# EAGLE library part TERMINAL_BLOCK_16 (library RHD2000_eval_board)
16-point terminal block
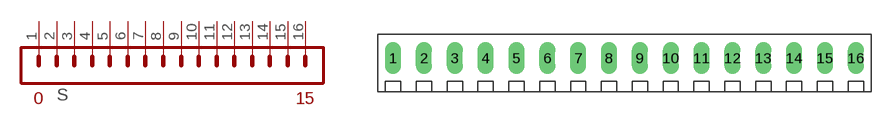
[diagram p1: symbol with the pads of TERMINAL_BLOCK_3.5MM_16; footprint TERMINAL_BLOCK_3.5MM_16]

Designator prefix S

## TERMINAL_BLOCK_16-3.5MM  [TERMINAL_BLOCK_3.5MM_16]
1  0  pas
2  1  pas
3  2  pas
4  3  pas
5  4  pas
6  5  pas
7  6  pas
8  7  pas
9  8  pas
10  9  pas
11  10  pas
12  11  pas
13  12  pas
14  13  pas
15  14  pas
16  15  pas

## Footprint TERMINAL_BLOCK_3.5MM_16 (pad centres in mm)
drill 1.2 long: 1 -26.25,0; 2 -22.75,0; 3 -19.25,0; 4 -15.75,0; 5 -12.25,0; 6 -8.75,0; 7 -5.25,0; 8 -1.75,0; 9 1.75,0; 10 5.25,0; 11 8.75,0; 12 12.25,0; 13 15.75,0; 14 19.25,0; 15 22.75,0; 16 26.25,0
